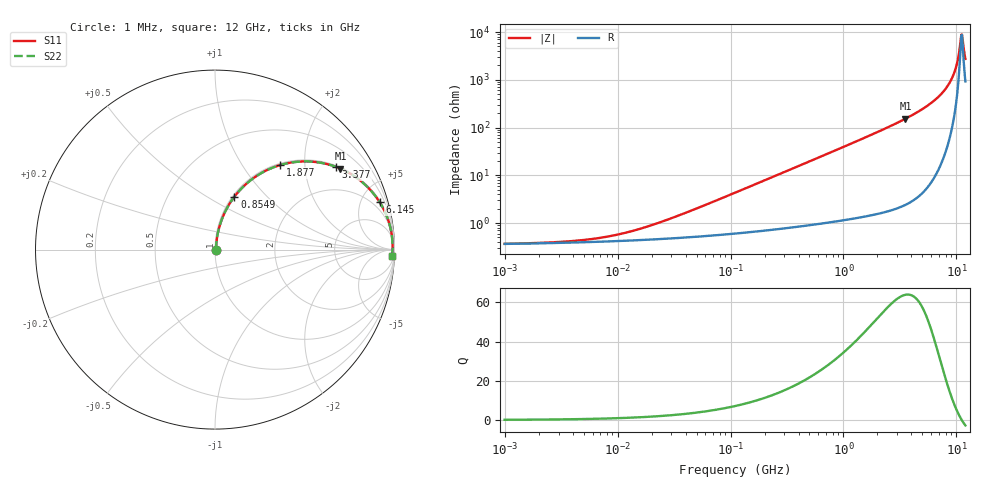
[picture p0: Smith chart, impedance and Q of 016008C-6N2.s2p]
# MHz S MA R 50
!Freq  MagS11  AngS11  MagS21  AngS21  MagS12  AngS12  MagS22  AngS22
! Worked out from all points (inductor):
!   801 points, 1 MHz to 12 GHz, reference 50 ohm
!   read as one part in series: L = 6.2 nH near 38.08 MHz
!   highest Q = 63.8 at 3.539 GHz (marker M1), where L = 6.9 nH
!   self-resonance near 11.05 GHz
!   S11 on the Smith chart (normalised r, x): 1 MHz: 1.01, +0.00; 854.9 MHz: 1.02, +0.67; 1.877 GHz: 1.03, +1.51; 3.377 GHz: 1.05, +2.90; 6.145 GHz: 1.16, +6.89; 12 GHz: 20, -51
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1  0.003656 6.1  0.9964 -0.0  0.9964 -0.0  0.003656 6.1
4.822396  0.004354 25.3  0.9961 -0.1  0.9961 -0.1  0.004354 25.3
10.46635  0.005833 43.9  0.9958 -0.2  0.9958 -0.2  0.005833 43.9
22.98406  0.01002 62.3  0.9954 -0.5  0.9954 -0.5  0.01002 62.3
110.8382  0.0433 79.6  0.9931 -2.5  0.9931 -2.5  0.0433 79.6
261.1649  0.1008 80.1  0.9876 -5.8  0.9876 -5.8  0.1008 80.1
528.267  0.2004 75.9  0.9709 -11.6  0.9709 -11.6  0.2004 75.9
854.8925  0.3148 69.8  0.9391 -18.3  0.9391 -18.3  0.3148 69.8
1274.315  0.445 62.2  0.8845 -26.4  0.8845 -26.4  0.445 62.2
1877.34  0.5958 52.3  0.7914 -36.6  0.7914 -36.6  0.5958 52.3
2517.778  0.7127 43.6  0.6893 -45.4  0.6893 -45.4  0.7127 43.6
3376.695  0.817 34.3  0.5639 -54.8  0.5639 -54.8  0.817 34.3
3539.058  0.8318 32.8  0.5423 -56.3  0.5423 -56.3  0.8318 32.8
4802.43  0.9114 23.4  0.3964 -65.7  0.3964 -65.7  0.9114 23.4
6145.25  0.9545 16.1  0.2772 -72.6  0.2772 -72.6  0.9545 16.1
7681.042  0.9783 9.9  0.1714 -77.8  0.1714 -77.8  0.9783 9.9
9053.277  0.9873 5.4  0.09516 -79.6  0.09516 -79.6  0.9873 5.4
9944.836  0.9895 3.0  0.05246 -76.9  0.05246 -76.9  0.9895 3.0
10796.69  0.9895 0.8  0.0175 -52.9  0.0175 -52.9  0.9895 0.8
11053.21  0.9893 0.2  0.01126 -17.4  0.01126 -17.4  0.9893 0.2
11449.47  0.9886 -0.7  0.01697 47.4  0.01697 47.4  0.9886 -0.7
12000  0.9872 -1.9  0.03609 68.3  0.03609 68.3  0.9872 -1.9
